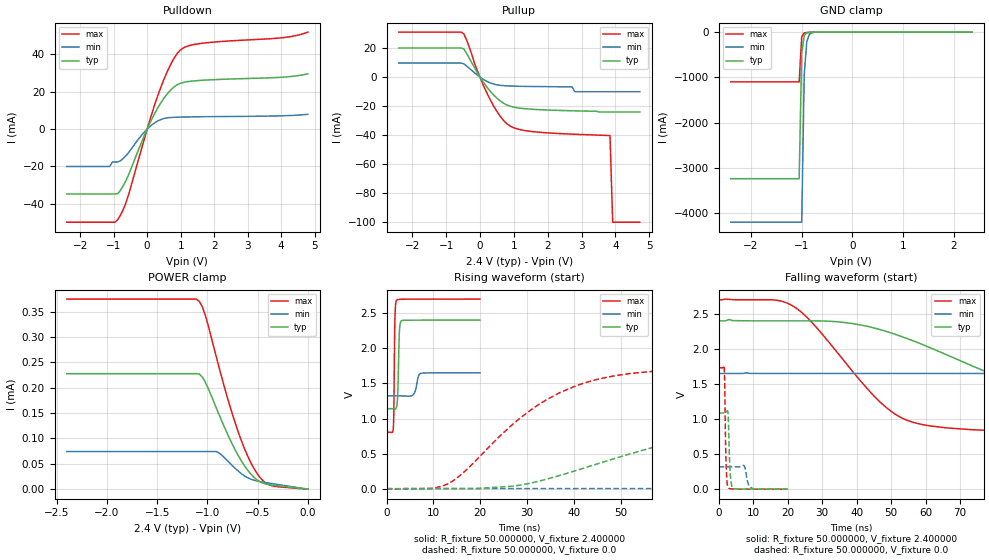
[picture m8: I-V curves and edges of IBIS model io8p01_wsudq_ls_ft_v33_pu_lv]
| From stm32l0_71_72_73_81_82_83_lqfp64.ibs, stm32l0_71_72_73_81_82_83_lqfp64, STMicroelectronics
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|   Model io8p01_wsudq_ls_ft_v33_pu_lv
[Model]  io8p01_wsudq_ls_ft_v33_pu_lv
Model_type I/O
Polarity   Non-Inverting
Enable   Active-Low
Vinl =   0.720000V
Vinh =   1.680000V
Vmeas =  1.200000V
Cref =   50.000000pF
Rref =   100.000000M
Vref =   0.0V
C_comp   2.582000pF   2.574200pF   2.601000pF
[Temperature Range]   25.000000   0.105000k   -40.000000
[Pullup Reference]   2.400000V   1.650000V   2.700000V
[Pulldown Reference]   0.0V   0.0V   0.0V
[POWER Clamp Reference]   2.400000V   1.650000V   2.700000V
[GND Clamp Reference]   0.0V   0.0V   0.0V
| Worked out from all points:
|   slope of the pulldown table from 0 to 0.36 V, typ, clamps not added: 28.5 ohm
|   slope of the pullup table from 0 to 0.36 V, typ, clamps not added: 32.2 ohm
|   GND clamp passes 1 mA (typ) near -0.65 V on its own axis
|   rising waveform, R_fixture 50.000000, V_fixture 2.400000: 20-80 % time 278ps typ, 628ps min, 192ps max; typ from 1.14 V to 2.4 V
|   rising waveform, R_fixture 50.000000, V_fixture 0.0: 20-80 % time 39.6ns typ, 107ns min, 19.4ns max; typ from 0.001 V to 1.09 V
|   falling waveform, R_fixture 50.000000, V_fixture 2.400000: 20-80 % time 41ns typ, 104ns min, 20.1ns max; typ from 2.4 V to 1.14 V
|   falling waveform, R_fixture 50.000000, V_fixture 0.0: 20-80 % time 477ps typ, 844ps min, 380ps max; typ from 1.09 V to 0.001 V
[Pulldown]
|Voltage   I(typ)   I(min)   I(max)
-2.4V     -34.71mA   -20mA      -49.82mA
-1.12V    -34.71mA   -20mA      -49.82mA
-1.04V    -34.71mA   -17.61mA   -49.82mA
-880mV    -34.55mA   -17.61mA   -48.46mA
-560mV    -24.65mA   -12.68mA   -35.33mA
0V        0A         0A         0A
400mV     13.84mA    5.066mA    22.03mA
720mV     21.25mA    6.254mA    35.26mA
1.04V     24.83mA    6.464mA    43.02mA
1.6V      26.11mA    6.627mA    45.88mA
4V        27.76mA    7.125mA    48.88mA
4.8V      29.64mA    7.94mA     51.96mA
[Pullup]
|Voltage   I(typ)   I(min)   I(max)
-2.4V     20.17mA    9.812mA    31.12mA
-480mV    19.53mA    9.213mA    29.94mA
0V        -580fA     6.14pA     10fA
320mV     -10.16mA   -4.078mA   -16.34mA
640mV     -17.08mA   -5.718mA   -28.28mA
960mV     -20.45mA   -6.129mA   -34.49mA
1.76V     -22.39mA   -6.471mA   -37.97mA
2.72V     -23.16mA   -6.63mA    -39.27mA
2.8V      -23.2mA    -10mA      -39.35mA
3.84V     -24mA      -10mA      -40.2mA
3.92V     -24mA      -10mA      -100mA
4.72V     -24mA      -10mA      -100mA
[GND_clamp]
|Voltage   I(typ)   I(min)   I(max)
-2.4V     -3.237A    -4.198A    -1.1A
-1.05V    -3.237A    -4.198A    -1.1A
-1V       -475.9mA   -4.198A    -104.3mA
-950mV    -76.36mA   -935.5mA   -18.56mA
-900mV    -16.77mA   -213mA     -9.293mA
-850mV    -6.713mA   -51.08mA   -6.724mA
-800mV    -4.108mA   -13.94mA   -4.924mA
-650mV    -1.048mA   -1.2mA     -1.149mA
2.35V     0A         0A         0A
[POWER_clamp]
|Voltage   I(typ)   I(min)   I(max)
-2.4V     228uA      74.29uA    375.2uA
-1.11V    228uA      74.29uA    375.2uA
-1.08V    227.1uA    74.29uA    370.5uA
-1.02V    210.9uA    74.29uA    342.6uA
-900mV    154.7uA    73.58uA    252.2uA
-810mV    113.1uA    58.15uA    186.8uA
-720mV    76.17uA    40.44uA    128.5uA
-630mV    45.92uA    26.04uA    79.56uA
-540mV    23.97uA    17.88uA    41.93uA
-450mV    12.07uA    14.02uA    17.32uA
-390mV    9.04uA     12.05uA    8.867uA
0V        0A         0A         0A
[Ramp]
| variable   typ   min   max
dV/dt_r  0.65095/39.55269n   0.19019/0.10658u   1.03799/19.31110n
dV/dt_f  0.75618/40.93497n   0.19440/0.10435u   1.13779/20.05602n
R_load = 50.000000
[Rising Waveform]
R_fixture= 50.000000
V_fixture= 2.400000
V_fixture_min= 1.650000
V_fixture_max= 2.700000
|time   V(typ)   V(min)   V(max)
0s        1.14V      1.323V     803.7mV
1.401ns   1.137V     1.323V     853mV
1.522ns   1.135V     1.323V     1.09V
1.762ns   1.132V     1.323V     2.415V
2.122ns   1.168V     1.323V     2.683V
2.362ns   1.347V     1.323V     2.693V
2.723ns   2.246V     1.323V     2.696V
3.083ns   2.385V     1.322V     2.697V
7.247ns   2.4V       1.641V     2.7V
19.94ns   2.4V       1.65V      2.7V
[Rising Waveform]
R_fixture= 50.000000
V_fixture= 0.0
V_fixture_min= 0.0
V_fixture_max= 0.0
|time   V(typ)   V(min)   V(max)
0s        880.8uV    1.332mV    514.1uV
13.01ns   2.447mV    2.47mV     66.78mV
29.03ns   57.58mV    2.472mV    1.031V
38.04ns   209.6mV    2.472mV    1.397V
47.05ns   396.1mV    2.484mV    1.586V
60.06ns   641.3mV    2.542mV    1.687V
89.09ns   952.5mV    4.355mV    1.727V
132.1ns   1.069V     62.37mV    1.73V
258.3ns   1.086V     273.4mV    1.73V
498.5ns   1.086V     318.6mV    1.73V
[Falling Waveform]
R_fixture= 50.000000
V_fixture= 2.400000
V_fixture_min= 1.650000
V_fixture_max= 2.700000
|time   V(typ)   V(min)   V(max)
0s        2.4V       1.65V      2.7V
21.02ns   2.4V       1.65V      2.626V
27.03ns   2.4V       1.65V      2.378V
49.05ns   2.242V     1.65V      1.147V
56.06ns   2.121V     1.65V      958.5mV
66.07ns   1.917V     1.65V      874.1mV
97.1ns    1.374V     1.65V      816.6mV
133.1ns   1.206V     1.639V     805.9mV
281.3ns   1.14V      1.388V     803.7mV
498.5ns   1.14V      1.323V     803.7mV
[Falling Waveform]
R_fixture= 50.000000
V_fixture= 0.0
V_fixture_min= 0.0
V_fixture_max= 0.0
|time   V(typ)   V(min)   V(max)
0s        1.086V     318.6mV    1.73V
1.642ns   1.086V     318.6mV    1.731V
2.162ns   1.088V     318.6mV    379.8mV
2.402ns   1.108V     318.6mV    121.1mV
2.763ns   1.047V     318.6mV    25.64mV
3.283ns   290.9mV    318.6mV    7.192mV
4.004ns   21.57mV    318.6mV    3.959mV
7.367ns   1.531mV    334.9mV    723uV
10.13ns   1mV        6.522mV    584.9uV
19.94ns   880.8uV    1.332mV    514.1uV
